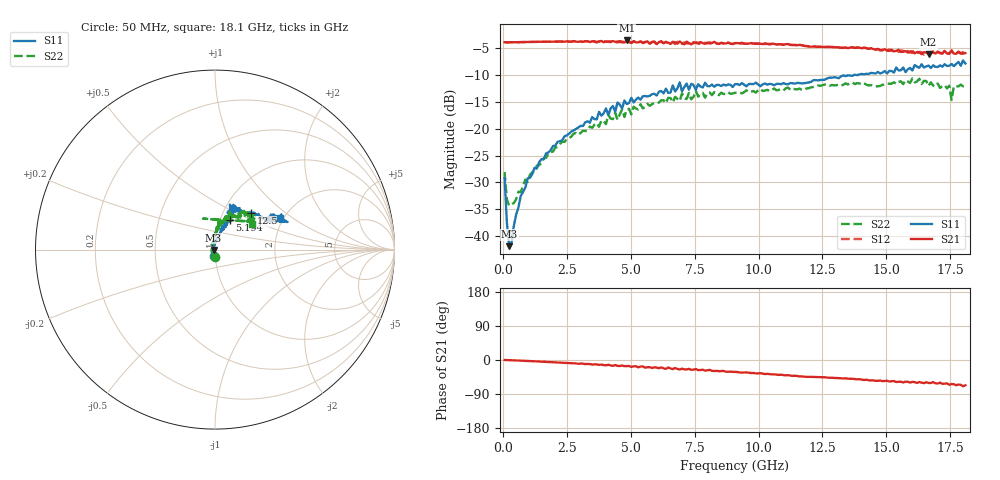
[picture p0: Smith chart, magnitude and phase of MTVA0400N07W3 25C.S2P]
! Network Analyzer HP8720D.06.14 Serial No. US36140669
!  8 Jul 2005  07:14:48
! Frequency  S11  S21  S12  S22
# HZ  S  DB R 50
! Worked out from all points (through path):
!   201 points, 50 MHz to 18.1 GHz, reference 50 ohm
!   highest |S21| = -3.56 dB at 4.833 GHz (marker M1); lowest = -6.1 dB at 16.66 GHz (marker M2)
!   group delay of S21, straight-line fit = 10.5 ps
!   lowest |S11| = -41.9 dB at 230.5 MHz (marker M3), VSWR 1.02, Z = 49.2 - j0.231 ohm
!   |S11| at or under -10 dB: start of sweep to 13.74 GHz; 13.83576 GHz to 13.87387 GHz (38.11 MHz wide, 0.275 % of centre)
!   |S22| runs from -34.3 to -10.6 dB; largest |S21 - S12| = 0.52
!   S11 on the Smith chart (normalised r, x): 50 MHz: 0.99, -0.07; 5.194 GHz: 1.11, +0.38; 12.5 GHz: 1.35, +0.60; 18.1 GHz: 1.92, +0.81
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5e7  -29.17 -96.3  -3.89 0.1  -3.90 0.2  -28.06 -93.2
1.4025e8  -37.57 -122.0  -3.94 -0.2  -3.92 -0.2  -33.23 -146.0
2.305e8  -41.87 -163.1  -3.91 -0.3  -3.90 -0.4  -34.33 -171.6
6.8175e8  -32.52 101.3  -3.87 -1.8  -3.87 -1.7  -31.79 130.7
9.525e8  -29.24 91.3  -3.84 -2.5  -3.84 -2.4  -29.92 116.9
1.76475e9  -24.42 81.2  -3.77 -5.2  -3.79 -5.4  -24.65 94.8
3.1185e9  -19.50 72.2  -3.81 -9.5  -3.83 -10.0  -20.37 88.3
4.83325e9  -15.40 72.5  -3.56 -16.1  -3.84 -17.1  -16.39 73.3
5.19425e9  -14.58 63.8  -3.92 -16.5  -3.73 -16.9  -16.25 82.1
6.09675e9  -13.09 65.4  -3.87 -21.6  -3.77 -21.1  -15.11 72.2
6.909e9  -11.37 67.7  -3.75 -25.3  -3.89 -23.1  -14.84 66.0
6.99925e9  -13.05 68.0  -4.06 -22.9  -4.23 -25.3  -13.40 66.4
7.17975e9  -11.58 71.8  -3.78 -24.9  -4.11 -23.3  -14.47 62.0
9.075e9  -11.70 63.0  -4.07 -31.4  -4.04 -31.5  -13.30 59.2
1.21435e10  -10.98 47.3  -4.68 -44.5  -4.63 -44.5  -12.23 56.0
1.25045e10  -10.89 45.7  -4.75 -45.4  -4.80 -45.8  -11.90 53.6
1.512175e10  -9.20 27.6  -5.48 -56.9  -5.22 -56.3  -11.61 49.6
1.6656e10  -8.24 27.9  -6.14 -60.6  -5.93 -58.4  -12.04 37.8
1.746825e10  -8.27 24.0  -6.04 -65.4  -5.99 -65.1  -11.99 38.8
1.75585e10  -7.94 22.9  -5.53 -63.5  -5.37 -5.6  -14.66 111.2
1.764875e10  -8.34 26.0  -6.02 -64.0  -5.99 -65.4  -12.07 38.8
1.81e10  -7.85 25.9  -5.92 -66.7  -6.26 -67.0  -12.01 35.1
